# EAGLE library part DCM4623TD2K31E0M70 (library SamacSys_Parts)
Isolated DC/DC Converters 500W 270Vin 28Vout 4623 Package Source: Datasheet
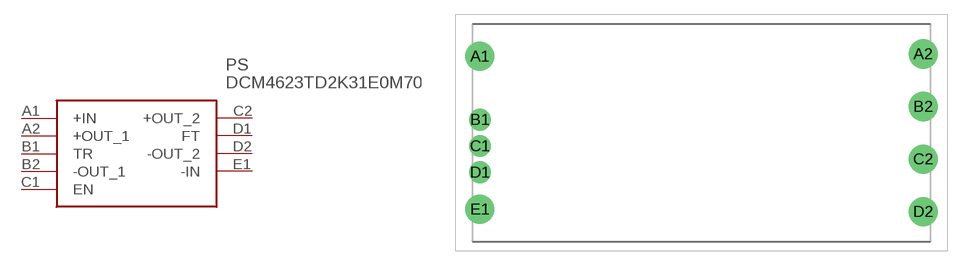
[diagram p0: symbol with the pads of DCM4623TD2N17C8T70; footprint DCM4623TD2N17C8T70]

Designator prefix PS

## DCM4623TD2K31E0M70 (Description: Isolated DC/DC Converters 500W 270Vin 28Vout 4623 Package; Height: 5mm; Manufacturer_Name: VICOR; Manufacturer_Part_Number: DCM4623TD2K31E0M70; Mouser_Part_Number: 492-DCM4623D2K31E0M7; Mouser_Price-Stock: https://www.mouser.com/Search/Refine.aspx?Keyword=492-DCM4623D2K31E0M7)  [DCM4623TD2N17C8T70]
A1  +IN
A2  +OUT_1
B1  TR
B2  -OUT_1
C1  EN
C2  +OUT_2
D1  FT
D2  -OUT_2
E1  -IN

## Footprint DCM4623TD2N17C8T70 (pad centres in mm)
DCM4623xD2N17C8y7z
drill 2.03 pad 3.045: A1 -23.19,8; A2 23.19,8.25; B2 23.19,2.75; C2 23.19,-2.75; D2 23.19,-8.25; E1 -23.19,-8
drill 1.52 pad 2.28: B1 -23.19,1.38; C1 -23.19,-1.38; D1 -23.19,-4.14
